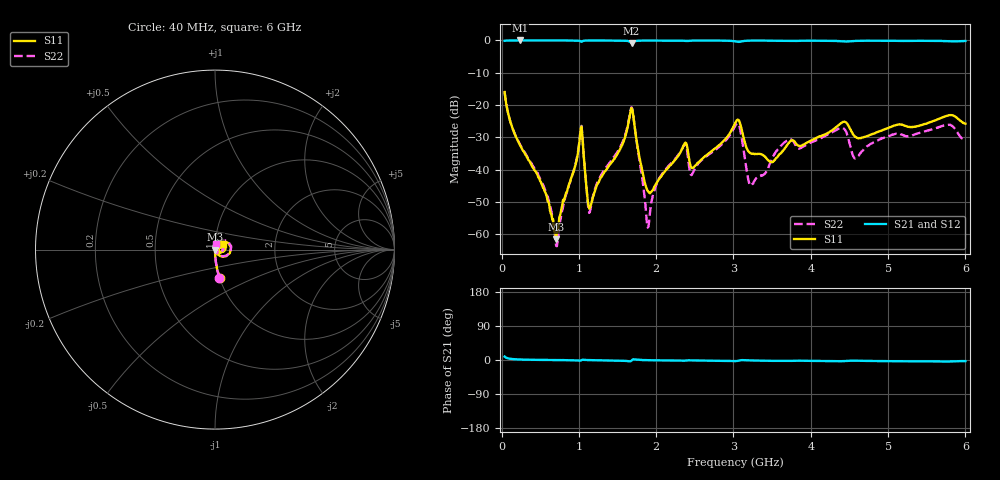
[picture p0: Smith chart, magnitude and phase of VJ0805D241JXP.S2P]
! VJ0805D241JXP
! DATE 03/14/2022  09:14
! CAPACITORS MOUNTED IN SERIES ON 25 MIL THICK MICROSTRIP SUBSTRATE
# GHz  S  MA  R  50.00
!  FREQ  S11M  S11A  S21M  S21A  S12M  S12A  S22M  S22A
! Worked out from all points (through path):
!   600 points, 40 MHz to 6 GHz, reference 50 ohm
!   highest |S21| = 0.00 dB at 239 MHz (marker M1); lowest = -0.8 dB at 1.682 GHz (marker M2)
!   lowest |S11| = -61.6 dB at 706.6 MHz (marker M3), VSWR 1.00, Z = 50.1 - j0.00277 ohm
!   |S11| at or under -10 dB: start of sweep to end of sweep
!   |S22| runs from -63.7 to -15.9 dB; largest |S21 - S12| = 0.0043
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0.04  0.1586 -80.6  0.9873 9.0  0.9862 9.1  0.1607 -81.2
0.239  0.02396 -88.5  0.9999 1.3  0.9996 1.3  0.02442 -88.4
0.56735  0.004418 -80.8  0.9991 0.1  0.9999 0.1  0.004697 -84.1
0.70665  0.0008329 -1.9  0.9995 -0.2  1 -0.2  0.0006567 -25.3
1.035  0.04621 -3.5  0.9538 -0.2  0.954 -0.2  0.04747 0.3
1.14445  0.002565 16.9  0.9983 -0.4  0.999 -0.4  0.002255 32.1
1.68175  0.08966 7.3  0.9108 -1.5  0.9117 -1.5  0.09237 11.7
1.8907  0.004688 -16.2  0.9975 -0.5  0.9981 -0.5  0.001266 8.6
2.03  0.006892 46.4  0.9975 -0.9  0.9986 -0.9  0.006921 88.9
2.35835  0.02399 44.9  0.988 -1.8  0.9889 -1.8  0.02351 69.5
2.4678  0.01051 28.3  0.9945 -1.1  0.9957 -1.1  0.00862 68.3
3.025  0.05326 34.1  0.9674 -2.9  0.9687 -3.0  0.04799 53.7
3.0847  0.05249 -7.5  0.9556 -0.8  0.957 -0.9  0.04294 3.4
3.224  0.01792 -2.0  0.9948 -1.1  0.996 -1.2  0.005656 32.3
3.49265  0.0131 30.0  0.991 -2.2  0.992 -2.3  0.01429 115.3
3.6817  0.02289 54.8  0.9863 -2.3  0.9874 -2.3  0.0276 97.3
4.02  0.02883 50.9  0.9917 -2.3  0.993 -2.4  0.02677 92.3
4.40805  0.05385 37.1  0.9702 -3.1  0.971 -3.2  0.04419 62.1
4.58715  0.03158 22.2  0.9849 -1.8  0.9856 -1.9  0.01504 71.0
5.015  0.04474 45.8  0.9894 -3.1  0.9906 -3.1  0.03339 95.1
5.78115  0.06914 40.8  0.9739 -4.0  0.9756 -4.1  0.04928 78.2
6.00005  0.05133 35.2  0.9819 -3.0  0.9826 -3.1  0.02959 82.7
